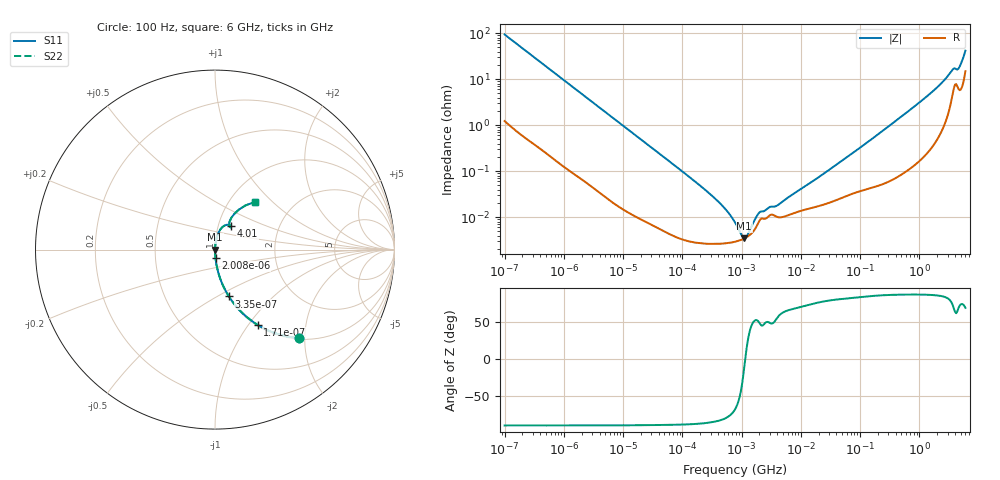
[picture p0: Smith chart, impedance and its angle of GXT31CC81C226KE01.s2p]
!Murata Part Number: GXT31CC81C226KE01
!These Parameters are Measured in Series Mode Connection
!Data Generated on Jan 08, 2026
!  o--ll--o
!Port1  Port2
!  o------o
!Operation Temp=25[degC], DC Bias Voltage=0[V]
!Freq. Start=100[Hz] Stop=6[GHz] 401[Steps]
# Hz S RI R 50
!Freq.(Hz) S11(Real) S11(Imag) S21(Real) S21(Imag) S12(Real) S12(Imag) S22(Real) S22(Imag)
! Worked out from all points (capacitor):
!   401 points, 100 Hz to 6 GHz, reference 50 ohm
!   read as one part in series: C = 16.8 uF near 109 Hz
!   lowest |Z| = 3.52 mohm at 1.108 MHz (marker M1)
!   series resonance near 1.153 MHz, so ESL is about 1.1 nH
!   S11 on the Smith chart (normalised r, x): 100 Hz: 1.02, -1.88; 171 Hz: 1.01, -1.11; 335 Hz: 1.01, -0.57; 2.008 kHz: 1.00, -0.10; 4.01 GHz: 1.15, +0.31; 6 GHz: 1.30, +0.78
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100  0.4707 -0.4926  0.5293 0.4926  0.5293 0.4926  0.4707 -0.4926
171  0.2369 -0.419  0.7631 0.419  0.7631 0.419  0.2369 -0.419
335  0.0774 -0.2609  0.9226 0.2609  0.9226 0.2609  0.0774 -0.2609
750  0.0176 -0.1252  0.9824 0.1252  0.9824 0.1252  0.0176 -0.1252
2008  0.00296 -0.0479  0.997 0.0479  0.997 0.0479  0.00296 -0.0479
40335  6.25e-05 -0.00245  0.9999 0.00245  0.9999 0.00245  6.25e-05 -0.00245
241822  2.68e-05 -0.000396  1 0.000396  1 0.000396  2.68e-05 -0.000396
432798  2.66e-05 -0.000199  1 0.000199  1 0.000199  2.66e-05 -0.000199
647581  2.8e-05 -0.000106  1 0.000106  1 0.000106  2.8e-05 -0.000106
774597  2.93e-05 -7.15e-05  1 7.15e-05  1 7.15e-05  2.93e-05 -7.15e-05
1108252  3.45e-05 -7e-06  1 7e-06  1 7e-06  3.45e-05 -7e-06
1658239  5.37e-05 6.81e-05  0.9999 -6.81e-05  0.9999 -6.81e-05  5.37e-05 6.81e-05
2967816  0.000109 0.000126  0.9999 -0.000126  0.9999 -0.000126  0.000109 0.000126
4060267  0.000101 0.000152  0.9999 -0.000152  0.9999 -0.000152  0.000101 0.000152
1.555665e7  0.000161 0.000573  0.9998 -0.000573  0.9998 -0.000573  0.000161 0.000573
3.124326e8  0.000698 0.00973  0.9993 -0.00973  0.9993 -0.00973  0.000698 0.00973
1.144649e9  0.00322 0.0356  0.9968 -0.0356  0.9968 -0.0356  0.00322 0.0356
2.240541e9  0.012 0.0751  0.988 -0.0751  0.988 -0.0751  0.012 0.0751
3.505958e9  0.0539 0.1343  0.9461 -0.1343  0.9461 -0.1343  0.0539 0.1343
4.009986e9  0.09 0.1308  0.91 -0.1308  0.91 -0.1308  0.09 0.1308
4.796499e9  0.0811 0.1556  0.9189 -0.1556  0.9189 -0.1556  0.0811 0.1556
6e9  0.2204 0.2651  0.7796 -0.2651  0.7796 -0.2651  0.2204 0.2651
